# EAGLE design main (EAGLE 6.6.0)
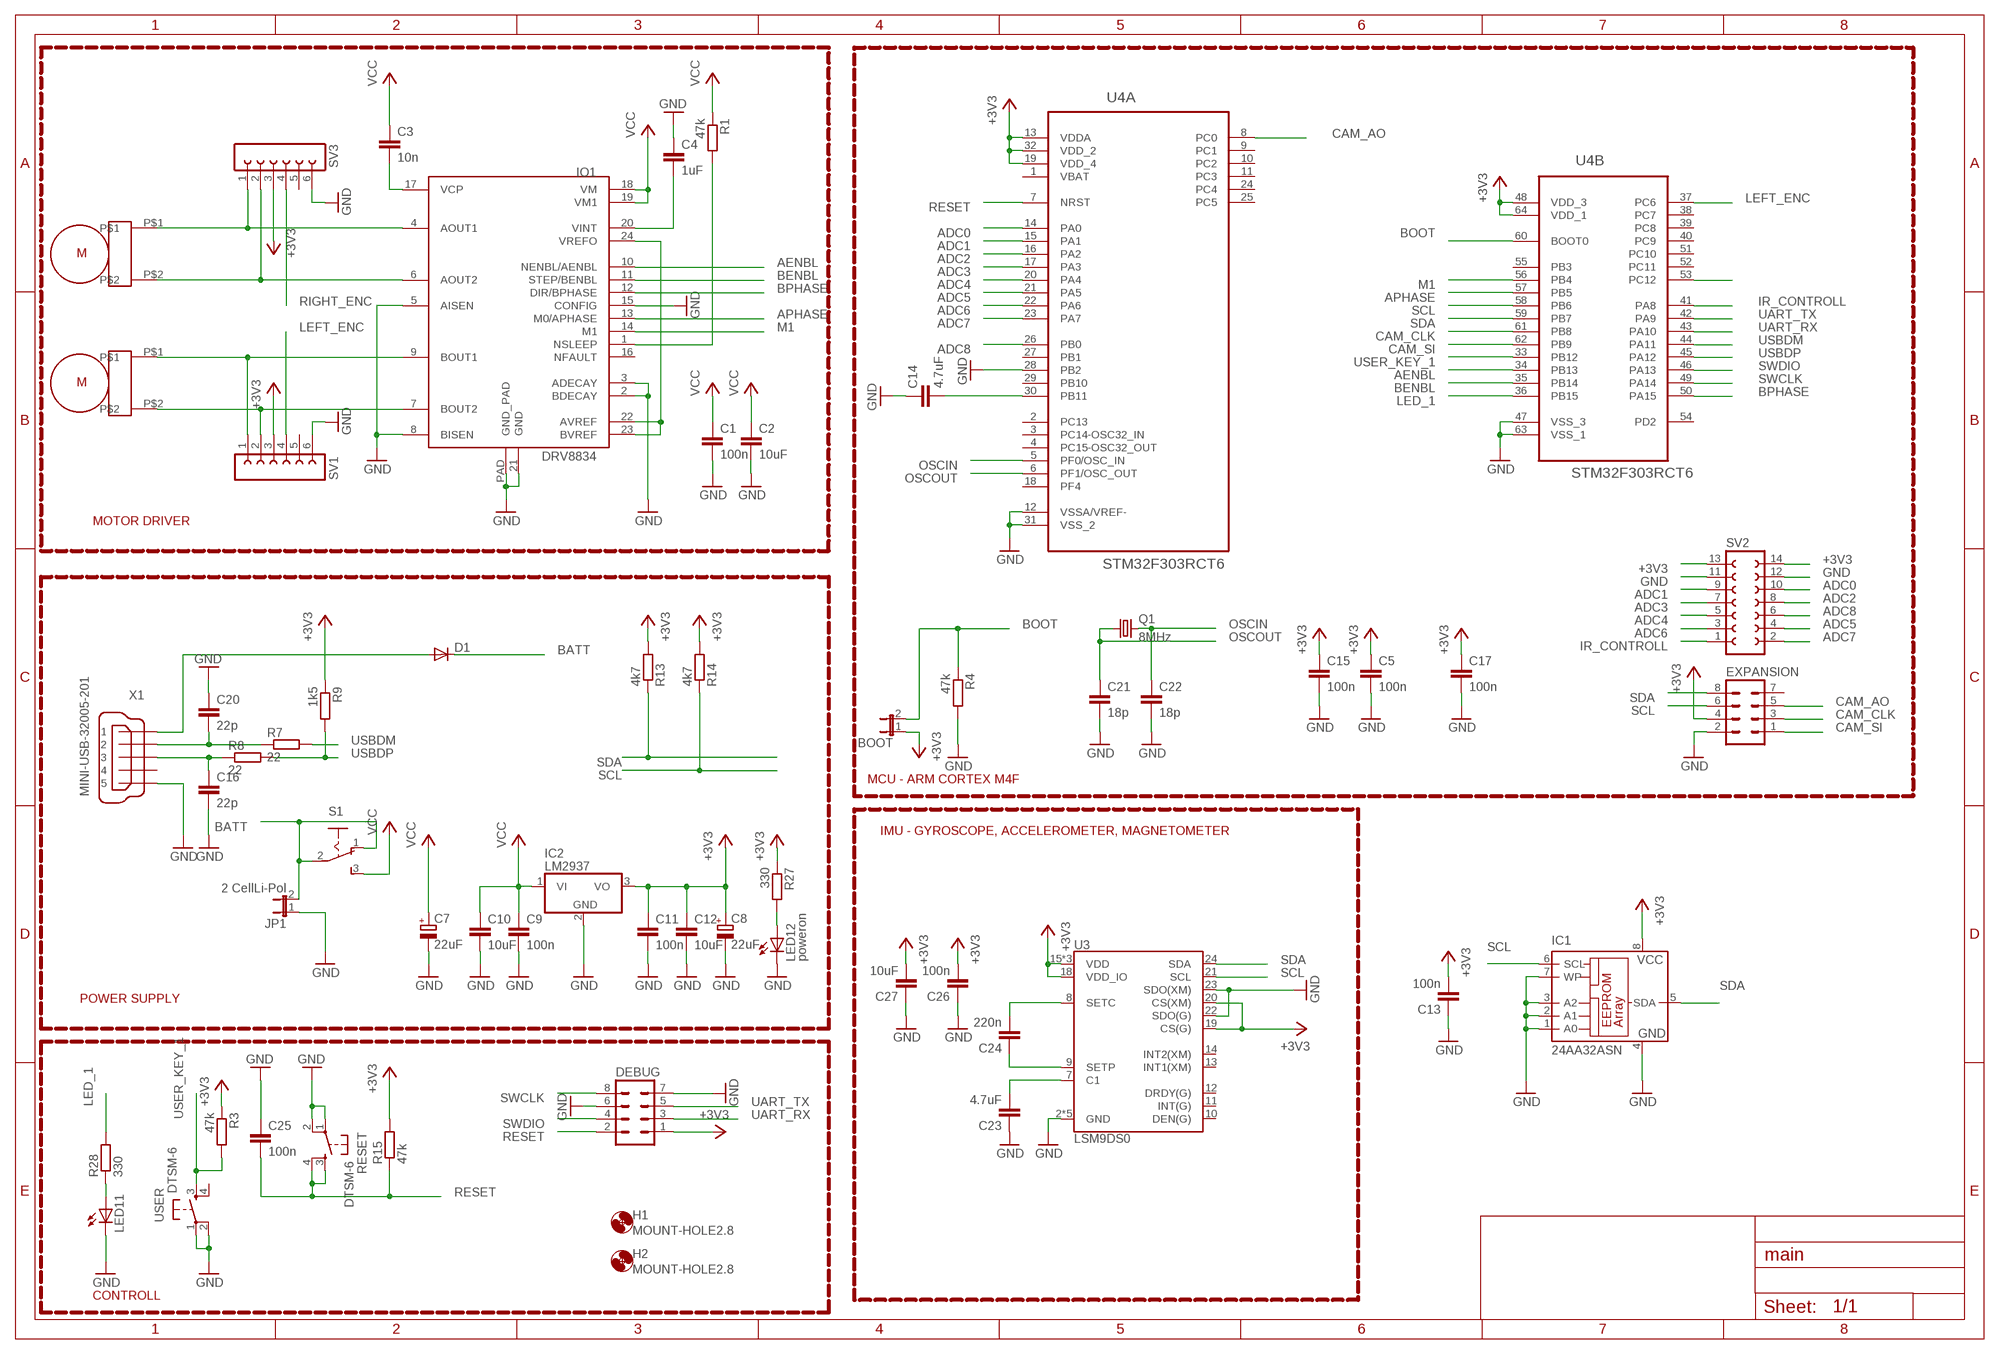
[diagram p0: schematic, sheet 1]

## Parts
BOOT  JP1E  [JP1]
C1  100n  C-EUC1206  [C1206]
C2  10uF  C-EUC1206  [C1206]
C3  10n  C-EUC1206  [C1206]
C4  1uF  C-EUC1206  [C1206]
C5  100n  C-EUC0805  [C0805]
C7  22uF  CPOL-EU153CLV-0505  [153CLV-0505]
C8  22uF  CPOL-EU153CLV-0505  [153CLV-0505]
C9  100n  C-EUC0805  [C0805]
C10  10uF  C-EUC0805  [C0805]
C11  100n  C-EUC0805  [C0805]
C12  10uF  C-EUC0805  [C0805]
C13  100n  C-EUC0805  [C0805]
C14  4.7uF  C-EUC0805  [C0805]
C15  100n  C-EUC0805  [C0805]
C16  22p  C-EUC0805  [C0805]
C17  100n  C-EUC0805  [C0805]
C20  22p  C-EUC0805  [C0805]
C21  18p  C-EUC0805  [C0805]
C22  18p  C-EUC0805  [C0805]
C23  4.7uF  C-EUC0805  [C0805]
C24  220n  C-EUC0805  [C0805]
C25  100n  C-EUC0805  [C0805]
C26  100n  C-EUC0805  [C0805]
C27  10uF  C-EUC0805  [C0805]
D1  DIODE-SMB  [SMB]
DEBUG  MA04-2  [MA04-2]
EXPANSION  MA04-2  [MA04-2]
H1  MOUNT-HOLE2.8  [2,8]
H2  MOUNT-HOLE2.8  [2,8]
IC1  24AA32ASN  [SO-08]
IC2  LM2937  [TO263-3]
IO1  DRV8834  [DRV8834_PCK]
JP1  2 CellLi-Pol  JP1E  [JP1]
LED11  LEDCHIPLED_1206  [CHIPLED_1206]
LED12  poweron  LEDCHIPLED_1206  [CHIPLED_1206]
Q1  8MHz  CRYSTALCTS406  [CTS406]
R1  47k  R-EU_M1206  [M1206]
R3  47k  R-EU_M0805  [M0805]
R4  47k  R-EU_M0805  [M0805]
R7  22  R-EU_M0805  [M0805]
R8  22  R-EU_M0805  [M0805]
R9  1k5  R-EU_M0805  [M0805]
R13  4k7  R-EU_M0805  [M0805]
R14  4k7  R-EU_M0805  [M0805]
R15  47k  R-EU_M0805  [M0805]
R27  330  R-EU_M0805  [M0805]
R28  330  R-EU_M0805  [M0805]
RESET  DTSM-6  [DTSM-6]
S1  255SB  [255SB]
SV1  FE06-1  [FE06]
SV2  FE07-2  [FE07-2]
SV3  FE06-1  [FE06]
U3  LSM9DS0  [LGA-24]
U4  STM32F303RCT6  [QFP50P1200X1200X160-64N]
U$1  MICRO_METAL_GEAR_MOTOR  [MICRO_METAL_GEAR_MOTOR]
U$2  MICRO_METAL_GEAR_MOTOR  [MICRO_METAL_GEAR_MOTOR]
USER  DTSM-6  [DTSM-6]
X1  MINI-USB-32005-201  [32005-201]

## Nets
+3V3: BOOT.1 C5.1 C8.+ C11.1 C12.1 C13.2 C15.1 C17.1 C26.2 C27.2 DEBUG.1 EXPANSION.4 IC1.8(VCC) IC2.3(VO) R3.1 R9.1 R13.2 R14.2 R15.2 R27.1 SV1.3 SV2.13 SV2.14 SV3.3 U3.15(VDD) U3.16(VDD) U3.17(VDD) U3.18(VDD_IO) U3.19(CS(G)) U3.20(CS(XM)) U4.13(A:VDDA) U4.19(A:VDD_4) U4.32(A:VDD_2) U4.48(B:VDD_3) U4.64(B:VDD_1)
ADC0: SV2.10 U4.14(A:PA0)
ADC1: SV2.9 U4.15(A:PA1)
ADC2: SV2.8 U4.16(A:PA2)
ADC3: SV2.7 U4.17(A:PA3)
ADC4: SV2.5 U4.20(A:PA4)
ADC5: SV2.4 U4.21(A:PA5)
ADC6: SV2.3 U4.22(A:PA6)
ADC7: SV2.2 U4.23(A:PA7)
ADC8: SV2.6 U4.26(A:PB0)
AENBL: IO1.10(NENBL/AENBL) U4.34(B:PB13)
APHASE: IO1.13(M0/APHASE) U4.57(B:PB5)
BATT: D1.C JP1.2 S1.1(O) S1.2(P)
BENBL: IO1.11(STEP/BENBL) U4.35(B:PB14)
BOOT: BOOT.2 R4.1 U4.60(B:BOOT0)
BPHASE: IO1.12(DIR/BPHASE) U4.50(B:PA15)
CAM_AO: EXPANSION.5 U4.8(A:PC0)
CAM_CLK: EXPANSION.3 U4.61(B:PB8)
CAM_SI: EXPANSION.1 U4.62(B:PB9)
GND: C1.2 C2.2 C4.1 C5.2 C7.- C8.- C9.2 C10.2 C11.2 C12.2 C13.1 C14.1 C15.2 C16.2 C17.2 C20.1 C21.2 C22.2 C23.1 C25.1 C26.1 C27.1 DEBUG.6 DEBUG.7 EXPANSION.2 IC1.1(A0) IC1.2(A1) IC1.3(A2) IC1.4(GND) IC1.7(WP) IC2.2(GND) IO1.2(BDECAY) IO1.3(ADECAY) IO1.5(AISEN) IO1.8(BISEN) IO1.15(CONFIG) IO1.21(GND) IO1.PAD(GND_PAD) JP1.1 LED11.C LED12.C R4.2 RESET.1 RESET.2 SV1.6 SV2.11 SV2.12 SV3.6 U3.2(GND) U3.3(GND) U3.4(GND) U3.5(GND) U3.6(GND) U3.22(SDO(G)) U3.23(SDO(XM)) U4.12(A:VSSA/VREF-) U4.28(A:PB2) U4.31(A:VSS_2) U4.47(B:VSS_3) U4.63(B:VSS_1) USER.1 USER.2 X1.5
IR_CONTROLL: SV2.1 U4.41(B:PA8)
LED_1: R28.2 U4.36(B:PB15)
LEFT_ENC: SV1.4 U4.37(B:PC6)
M1: IO1.14(M1) U4.56(B:PB4)
N$1: IO1.4(AOUT1) SV3.1 U$1.P$1
N$2: IO1.6(AOUT2) SV3.2 U$1.P$2
N$3: IO1.9(BOUT1) SV1.1 U$2.P$1
N$4: IO1.7(BOUT2) SV1.2 U$2.P$2
N$5: C3.2 IO1.17(VCP)
N$6: C23.2 U3.7(C1)
N$7: C24.2 U3.8(SETC)
N$8: IO1.22(AVREF) IO1.23(BVREF) IO1.24(VREFO)
N$9: IO1.1(NSLEEP) R1.2
N$13: C24.1 U3.9(SETP)
N$15: C14.2 U4.30(A:PB11)
N$22: C4.2 IO1.20(VINT)
N$23: LED12.A R27.2
N$33: LED11.A R28.1
N$55: C20.2 R7.1 X1.2
N$56: C16.1 R8.1 X1.3
N$57: D1.A X1.1
OSCIN: C22.1 Q1.3 U4.5(A:PF0/OSC_IN)
OSCOUT: C21.1 Q1.1 U4.6(A:PF1/OSC_OUT)
RESET: C25.2 DEBUG.2 R15.1 RESET.3 RESET.4 U4.7(A:NRST)
RIGHT_ENC: SV3.4 U4.53(B:PC12)
SCL: EXPANSION.6 IC1.6(SCL) R14.1 U3.21(SCL) U4.58(B:PB6)
SDA: EXPANSION.8 IC1.5(SDA) R13.1 U3.24(SDA) U4.59(B:PB7)
SWCLK: DEBUG.8 U4.49(B:PA14)
SWDIO: DEBUG.4 U4.46(B:PA13)
UART_RX: DEBUG.3 U4.43(B:PA10)
UART_TX: DEBUG.5 U4.42(B:PA9)
USBDM: R7.2 U4.44(B:PA11)
USBDP: R8.2 R9.2 U4.45(B:PA12)
USER_KEY_1: R3.2 U4.33(B:PB12) USER.3
VCC: C1.1 C2.1 C3.1 C7.+ C9.1 C10.1 IC2.1(VI) IO1.18(VM) IO1.19(VM1) R1.1 S1.3(S)
Unconnected: EXPANSION.7 IO1.16(NFAULT) SV1.5 SV3.5 U3.10(DEN(G)) U3.11(INT(G)) U3.12(DRDY(G)) U3.13(INT1(XM)) U3.14(INT2(XM)) U4.2(A:PC13) U4.3(A:PC14-OSC32_IN) U4.4(A:PC15-OSC32_OUT) U4.9(A:PC1) U4.10(A:PC2) U4.11(A:PC3) U4.18(A:PF4) U4.24(A:PC4) U4.25(A:PC5) U4.27(A:PB1) U4.29(A:PB10) U4.38(B:PC7) U4.39(B:PC8) U4.40(B:PC9) U4.51(B:PC10) U4.52(B:PC11) U4.54(B:PD2) U4.55(B:PB3) USER.4 X1.4

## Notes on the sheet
- MOTOR DRIVER
- MCU - ARM CORTEX M4F
- IMU - GYROSCOPE, ACCELEROMETER, MAGNETOMETER
- POWER SUPPLY
- CONTROLL

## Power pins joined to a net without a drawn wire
VBAT: U4.1(A:VBAT)

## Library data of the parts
BOOT JP1 = jumper:JP1E: JUMPER
C1-C5 C9-C17 C20-C27 = resistor:C-EU: CAPACITOR, European symbol
C7 C8 = resistor:CPOL-EU: POLARIZED CAPACITOR, European symbol
D1 = diode:DIODE-: DIODE
DEBUG EXPANSION = con-lstb:MA04-2: PIN HEADER; OC_FARNELL: unknown; OC_NEWARK: unknown
H1 H2 = holes:MOUNT-HOLE: MOUNTING HOLE with drill center marker
IC1 = microchip:24*: Serial EEPROM I2C; MF: MICROCHIP; MPN: 24AA32A-I/SN; OC_FARNELL: 1617659; OC_NEWARK: 83C5815
IC2 = linear:LM2937: LM2937-2.5, LM2937-3.3 400mA and 500mA Voltage Regulators Source: http://cache.national.com/ds/LM/LM2937-2.5.pdf
IO1 = yellow_car:DRV8834
LED11 LED12 = led:LED: LED
Q1 = crystal:CRYSTAL: CRYSTAL; OC_FARNELL: unknown; OC_NEWARK: unknown
R1 R3 R4 R7-R9 R13-R15 R27 R28 = resistor:R-EU_: RESISTOR, European symbol
RESET USER = switch-tact:DTSM-6
S1 = switch:255SB: SLIDING SWITCH Distributor Buerklin, 11G810
SV1 SV3 = con-lsta:FE06-1: FEMALE HEADER; OC_FARNELL: unknown; OC_NEWARK: unknown
SV2 = con-lsta:FE07-2: FEMALE HEADER; OC_FARNELL: unknown; OC_NEWARK: unknown
U3 = SparkFun-DigitalIC:LSM9DS0: LSM9DS0 3D Accelerometer, 3D Gyroscope, 3D Magnetomter Features: 3 acceleration channels, 3 angular rate channels, 3 magnetic field channels ±2/±4/±6/±8/±16 g linear acceleration full scale ±2/±4/±8/±12 gauss magnetic full scale ±245/±500/±2000 dps angular rate full scale 16-bit data output SPI /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
U4 = my_parts:STM32F303RCT6: ARM Cortex-M4 32b MCU+FPU,LQFP-64; MPN: STM32F303RCT6; OC_FARNELL: 2215112; OC_NEWARK: 46W2193; PACKAGE: LQFP-64; SUPPLIER: STMICROELECTRONICS
U$1 U$2 = pololu:MICRO_METAL_GEAR_MOTOR
X1 = con-cypressindustries:MINI-USB-: MINI USB-B Conector Source: www.cypressindustries.com; OC_FARNELL: unknown; OC_NEWARK: unknown

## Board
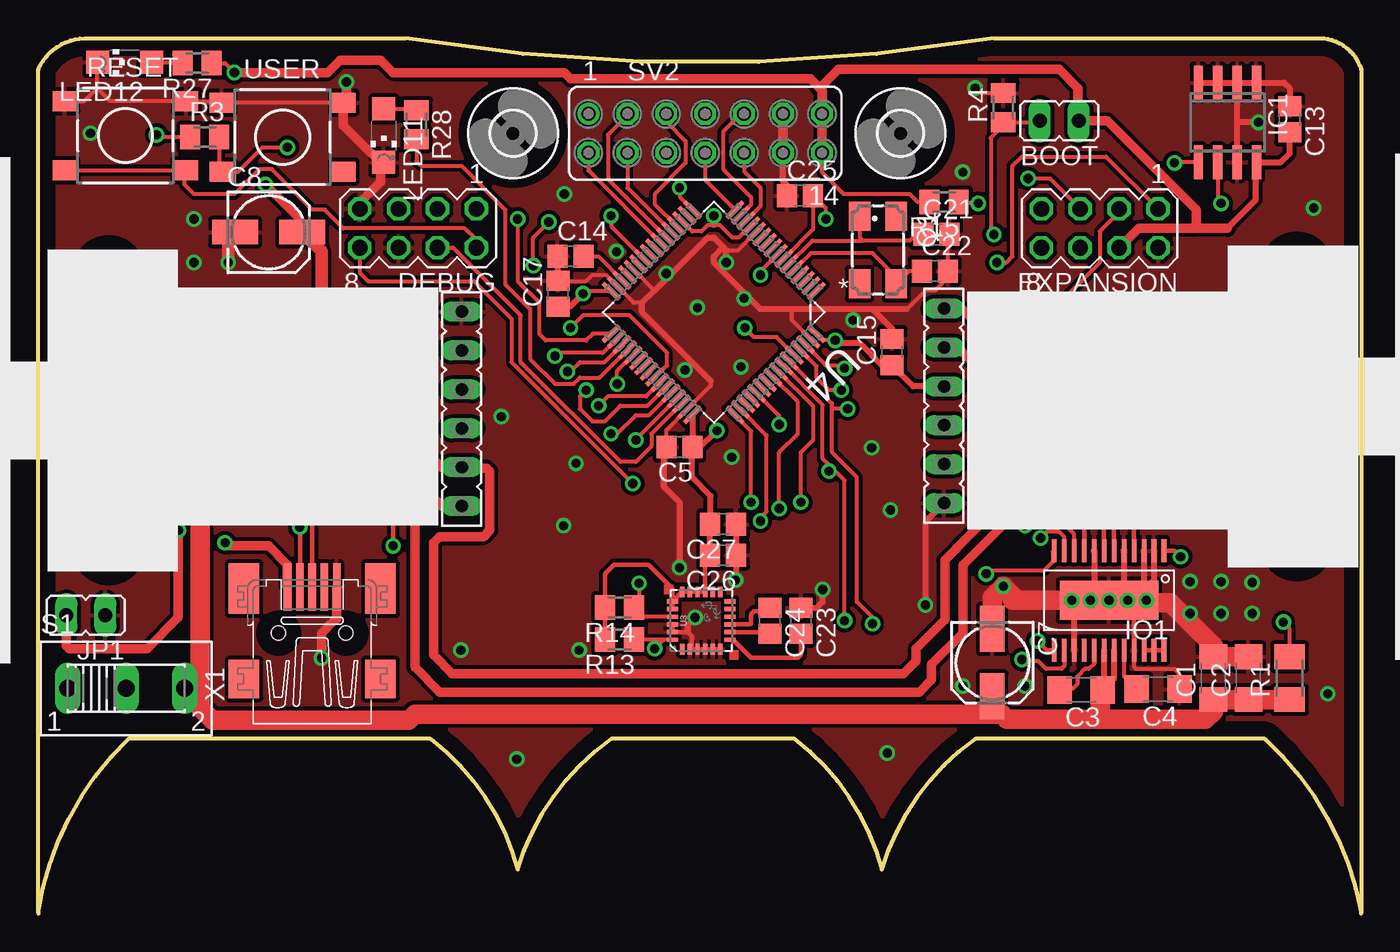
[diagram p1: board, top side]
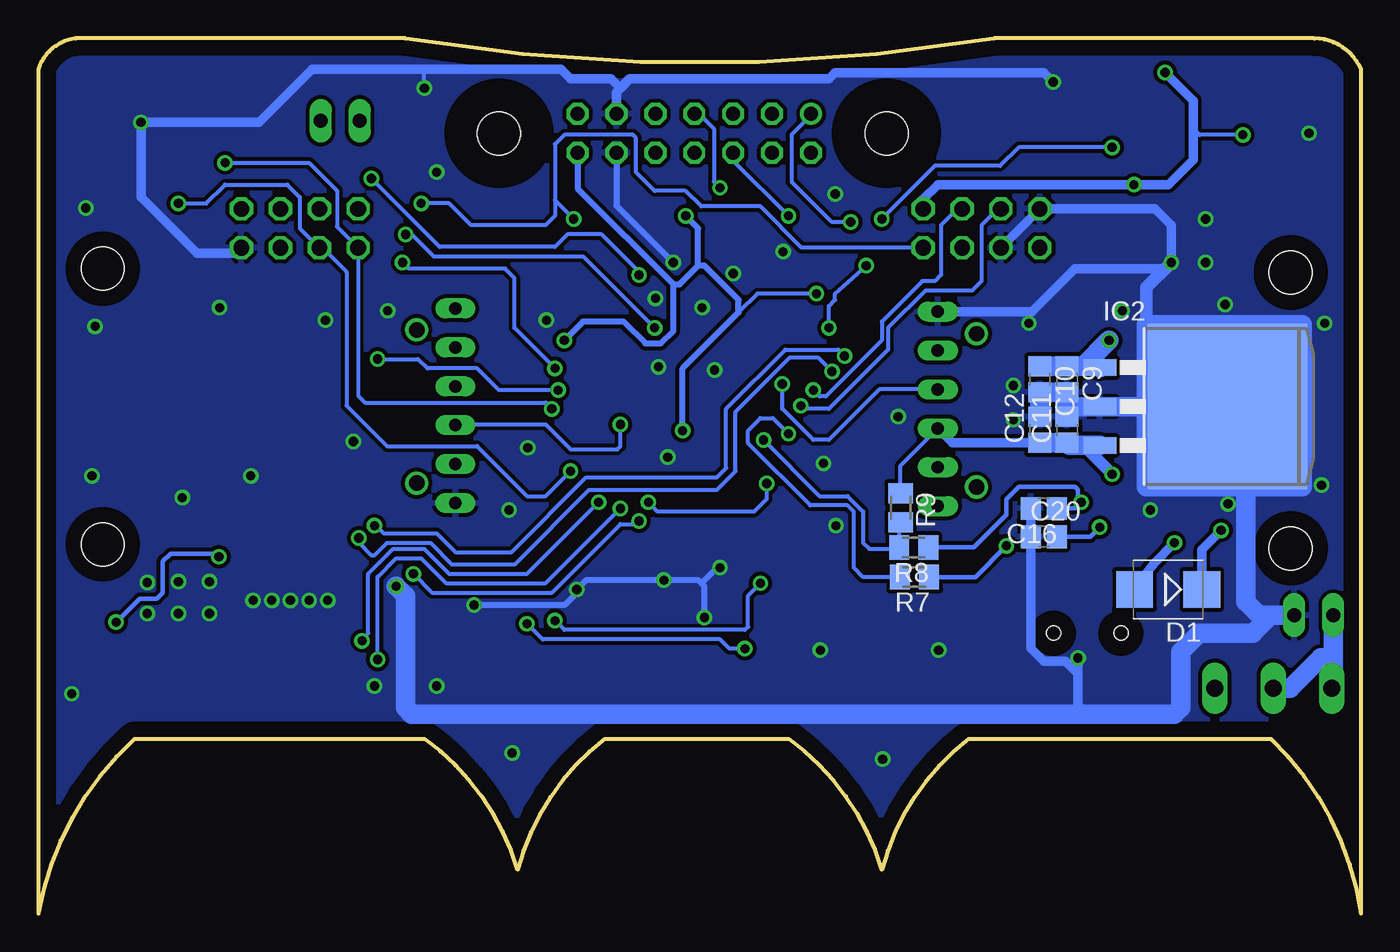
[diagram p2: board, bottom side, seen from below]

Size 86.36 x 57.1 mm. Coordinates in mm from the lower left corner, seen from the top.
Outline: 3.05,57.1 23.98,57.1 arc19 62.38,57.1 83.92,57.1 arc-66 86.36,55.07 86.36,0 arc38 80.06,11.38 61.16,11.38 arc38 55.07,2.85 arc38 49.38,11.38 37.39,11.38 arc38 31.29,2.85 arc38 25.6,11.38 5.89,11.38 arc38 0,0 0,55.07 arc-66 3.05,57.1
Copper layers (1*16): Top 0.035mm / dielectric 1.5mm / Bottom 0.035mm
Design rules "default *": minimum track width 10mil, minimum drill 24mil, track to track 10mil, track to pad 10mil, pad to pad 10mil, via to via 10mil, smd to smd 10mil, copper to edge 40mil, drill to drill 8mil, minimum pad ring 10mil, minimum via ring 8mil, stop-mask expansion 4mil, vias tented up to drill 0mil, thermal gap 10mil

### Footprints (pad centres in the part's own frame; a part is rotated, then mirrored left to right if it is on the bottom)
JP1 = drill 0.914 long: 1 0,-1.27; 2 0,1.27
C1206 = smd 1.6 x 1.8: 1 -1.4,0; 2 1.4,0
C0805 = smd 1.3 x 1.5: 1 -0.85,0; 2 0.85,0
153CLV-0505 = smd 3 x 1.6: + 2.2,0; - -2.2,0
SMB = smd 2.4 x 2.4: A 2.2,0; C -2.2,0
MA04-2 = drill 1.016 octagon: 1 -3.81,-1.27; 2 -3.81,1.27; 3 -1.27,-1.27; 4 -1.27,1.27; 5 1.27,-1.27; 6 1.27,1.27; 7 3.81,-1.27; 8 3.81,1.27
2,8 = hole 2.8: 0,0
SO-08 = smd 0.6 x 2.2: 1 -1.905,-2.6; 2 -0.635,-2.6; 3 0.635,-2.6; 4 1.905,-2.6; 5 1.905,2.6; 6 0.635,2.6; 7 -0.635,2.6; 8 -1.905,2.6
TO263-3 = smd 1.067 x 2.159: 1 -2.54,-5.791; 2 0,-5.791; 3 2.54,-5.791 | smd 10.8 x 10.41: TAB 0,2.54
DRV8834_PCK = smd 0.3 x 1.5: 1 -3.575,-3.25; 2 -2.925,-3.25; 3 -2.275,-3.25; 4 -1.625,-3.25; 5 -0.975,-3.25; 6 -0.325,-3.25; 7 0.325,-3.25; 8 0.975,-3.25; 9 1.625,-3.25; 10 2.275,-3.25; 11 2.925,-3.25; 12 3.575,-3.25; 13 3.575,3.25; 14 2.925,3.25; 15 2.275,3.25; 16 1.625,3.25; 17 0.975,3.25; 18 0.325,3.25; 19 -0.325,3.25; 20 -0.975,3.25; 21 -1.625,3.25; 22 -2.275,3.25; 23 -2.925,3.25; 24 -3.575,3.25 | smd 6.452 x 2.54: PAD 0,0
CHIPLED_1206 = smd 1.5 x 1.5: A 0,-1.75; C 0,1.75
CTS406 = smd 1.9 x 1.4: 1 -2.2,-1.2; 2 2.2,-1.2; 3 2.2,1.2; 4 -2.2,1.2
M1206 = smd 1.6 x 2: 1 -1.4,0; 2 1.4,0
M0805 = smd 1.3 x 1.6: 1 -0.95,0; 2 0.95,0
DTSM-6 = smd 1.55 x 1.3: 1 -3.975,2.25; 2 3.975,2.25; 3 -3.975,-2.25; 4 3.975,-2.25
255SB = drill 1.118 long: 1 -3.81,0; 2 0,0; 3 3.81,0
FE06 = drill 0.813 long: 1 -6.35,0; 2 -3.81,0; 3 -1.27,0; 4 1.27,0; 5 3.81,0; 6 6.35,0
FE07-2 = drill 0.914: 1 -7.62,1.27 | drill 0.914 octagon: 2 -7.62,-1.27; 3 -5.08,1.27; 4 -5.08,-1.27; 5 -2.54,1.27; 6 -2.54,-1.27; 7 0,1.27; 8 0,-1.27; 9 2.54,1.27; 10 2.54,-1.27; 11 5.08,1.27; 12 5.08,-1.27; 13 7.62,1.27; 14 7.62,-1.27
LGA-24 = smd 0.7 x 0.29: 1 -1.875,1.25; 2 -1.875,0.75; 3 -1.875,0.25; 4 -1.875,-0.25; 5 -1.875,-0.75; 6 -1.875,-1.25; 13 1.875,-1.25; 14 1.875,-0.75; 15 1.875,-0.25; 16 1.875,0.25; 17 1.875,0.75; 18 1.875,1.25 | smd 0.29 x 0.7: 7 -1.25,-1.875; 8 -0.75,-1.875; 9 -0.25,-1.875; 10 0.25,-1.875; 11 0.75,-1.875; 12 1.25,-1.875; 19 1.25,1.875; 20 0.75,1.875; 21 0.25,1.875; 22 -0.25,1.875; 23 -0.75,1.875; 24 -1.25,1.875
QFP50P1200X1200X160-64N = smd 1.473 x 0.279: 1 -5.715,3.759; 2 -5.715,3.251; 3 -5.715,2.743; 4 -5.715,2.261; 5 -5.715,1.753; 6 -5.715,1.245; 7 -5.715,0.762; 8 -5.715,0.254; 9 -5.715,-0.254; 10 -5.715,-0.762; 11 -5.715,-1.245; 12 -5.715,-1.753; 13 -5.715,-2.261; 14 -5.715,-2.743; 15 -5.715,-3.251; 16 -5.715,-3.759; 33 5.715,-3.759; 34 5.715,-3.251; 35 5.715,-2.743; 36 5.715,-2.261; 37 5.715,-1.753; 38 5.715,-1.245; 39 5.715,-0.762; 40 5.715,-0.254; 41 5.715,0.254; 42 5.715,0.762; 43 5.715,1.245; 44 5.715,1.753; 45 5.715,2.261; 46 5.715,2.743; 47 5.715,3.251; 48 5.715,3.759 | smd 0.279 x 1.473: 17 -3.759,-5.715; 18 -3.251,-5.715; 19 -2.743,-5.715; 20 -2.261,-5.715; 21 -1.753,-5.715; 22 -1.245,-5.715; 23 -0.762,-5.715; 24 -0.254,-5.715; 25 0.254,-5.715; 26 0.762,-5.715; 27 1.245,-5.715; 28 1.753,-5.715; 29 2.261,-5.715; 30 2.743,-5.715; 31 3.251,-5.715; 32 3.759,-5.715; 49 3.759,5.715; 50 3.251,5.715; 51 2.743,5.715; 52 2.261,5.715; 53 1.753,5.715; 54 1.245,5.715; 55 0.762,5.715; 56 0.254,5.715; 57 -0.254,5.715; 58 -0.762,5.715; 59 -1.245,5.715; 60 -1.753,5.715; 61 -2.261,5.715; 62 -2.743,5.715; 63 -3.251,5.715; 64 -3.759,5.715
MICRO_METAL_GEAR_MOTOR = drill 1: P$1 -5,1; P$2 5,1 | hole 2.8: -9,21.5; 9,21.5
32005-201 = smd 3.1 x 0.5: 1 3,1.6; 2 3,0.8; 3 3,0; 4 3,-0.8; 5 3,-1.6 | smd 2.5 x 2: M1 -3,-4.45; M2 -3,4.45 | smd 3.3 x 2: M3 2.9,4.45; M4 2.9,-4.45 | hole 0.9: 0,2.2; 0,-2.2

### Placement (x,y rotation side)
BOOT  66.65,51.71 90 top
C1  76.71,15.34 90 top
C2  78.99,15.34 90 top
C3  68.07,14.58 180 top
C4  73.1,14.63 180 top
C5  41.86,30.43 180 top
C7  62.28,16.36 270 top
C8  15.04,44.45 0 top
C9  19.2,34.85 270 bottom
C10  20.98,34.85 270 bottom
C11  19.2,31.55 90 bottom
C12  20.98,31.55 90 bottom
C13  81.69,51.82 270 top
C14  34.75,42.88 0 top
C15  55.73,36.63 90 top
C16  20.73,26.42 180 bottom
C17  33.93,40.44 90 top
C20  20.73,24.59 0 bottom
C21  58.62,44.3 0 top
C22  58.52,41.91 0 top
C23  49.78,19.1 270 top
C24  47.75,19.1 270 top
C25  49.73,46.84 0 top
C26  44.7,23.37 180 top
C27  44.7,25.4 180 top
D1  12.6,21.13 180 bottom
DEBUG  24.79,44.7 180 top
EXPANSION  69.29,44.7 180 top
H1  30.99,50.9 0 top
H2  56.29,50.9 0 top
IC1  77.62,51.61 180 top
IC2  11.28,33.07 270 bottom
IO1  69.9,20.42 180 top
JP1  3.1,19.46 90 top
LED11  22.56,50.75 180 top
LED12  5.64,55.52 90 top
Q1  54.81,43.28 270 top
R1  81.69,15.34 90 top
R3  10.87,50.65 0 top
R4  62.99,52.58 90 top
R7  29.16,21.95 180 bottom
R8  29.21,23.88 180 bottom
R9  30.07,26.47 270 bottom
R13  37.95,17.88 180 top
R14  37.95,19.96 180 top
R15  59.13,46.43 180 top
R27  10.36,55.47 180 top
R28  24.69,51.46 270 top
RESET  5.69,50.75 0 top
S1  5.74,14.68 0 top
SV1  27.64,32.92 90 top
SV2  43.54,50.9 0 top
SV3  59.13,33.12 270 top
U3  43.28,19.1 90 top
U4  44.09,39.22 225 top
U$1  60.66,33.07 270 top
U$2  26.11,32.82 90 top
USER  15.95,50.65 0 top
X1  17.88,18.29 90 top

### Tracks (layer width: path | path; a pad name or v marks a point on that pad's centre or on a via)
+3V3  (via drill 0.6)
  Top 0.254: R27.1 12.19,55.47 v12.8,54.86 | R3.1 7.87,50.65 v7.72,50.8 | C5.1 U4.48 | U4.13 46.48,44.86 45.72,44.09 45.31,44.09 44.5,44.91 44.09,44.91 43.69,44.91 43.28,44.5 42.69,44.5 U4.19 | R15.2 57.4,46.43 56.9,46.94 52.58,46.94 51.16,48.36 SV2.14 | U4.32 35.72,40.6 v35.56,40.44 | v52.02,37.39 51.24,37.39 U4.64
  Top 0.305: U3.20 U3.19 | U3.19 U3.18 U3.17 U3.16 U3.15 43.53,23.25 C26.2 | U3.19 41.41,21.18 39.83,22.76 37.59,22.76 36.98,22.15 36.98,19.98 R14.2 R13.2
  Top 0.406: C26.2 C27.2 43.89,25.44 43.89,27.23 42.67,28.45 42.67,30.28 | C13.2 81.69,49.58 81.12,49.01 IC1.8 79.45,48.94 79.45,46.53 77.62,44.7 | 42.67,30.28 42.67,30.39 C5.1 | U4.48 42.71,30.32 42.67,30.28 | 42.67,30.28 43.08,30.28 v44.3,31.5 | v44.09,45.52 44.09,44.91 | C17.1 34.71,39.59 v35.56,40.44 | SV3.3 57.11,34.39 C15.1 55.05,35.78 53.64,37.19 52.22,37.19 v52.02,37.39
  Top 0.61: C8.+ 17.07,44.62 17.07,45.31 v14.83,47.55 | v12.8,54.86 18.9,54.86 19.71,55.68 22.35,55.68 23.16,54.86 34.34,54.86 34.75,54.46 50.39,54.46 51.21,53.65 51.21,52.22 SV2.13 SV2.14 51.16,54 52.22,55.07 66.65,55.07 67.87,53.85 67.87,51.77 BOOT.1 69.8,51.71 75.59,45.92 75.59,44.91 75.39,44.7 | 75.39,44.7 71.83,44.7 EXPANSION.4 | 77.62,44.7 75.39,44.7
  Top 0.813: v16.26,28.65 16.26,34.54 18.49,36.78 18.49,43.2 C8.+
  Bottom 0.254: v7.72,50.8 10.57,50.8 10.97,51.21 | v35.56,40.44 39.42,40.44 40.64,39.22 | R9.1 30.07,29.21 SV1.3
  Bottom 0.406: SV2.14 51.16,47.3 44.91,41.05 | 44.91,41.05 44.5,41.05 43.28,42.27 | v44.3,31.5 44.3,35.56 40.64,39.22 40.64,40.03 42.88,42.27 43.28,42.27 | 43.28,42.27 43.28,44.7 v44.09,45.52 | 44.91,41.05 44.91,38 45.72,37.19 46.74,37.19 48.16,38.61 50.8,38.61 v52.02,37.39
  Bottom 0.61: DEBUG.1 28.6,46.58 27.63,47.55 v14.83,47.55 12.6,47.55 10.97,49.17 10.97,51.21 10.97,53.04 v12.8,54.86 | C12.1 26.68,30.7 SV1.3
  Bottom 0.813: C12.1 18.3,30.7 v16.26,28.65
  Bottom 1.27: IC2.3 19.04,30.53 C11.1 C12.1
ADC0
  Top 0.254: SV2.10 46.08,48.41 47.14,47.35 47.14,46.15 U4.14
ADC1
  Top 0.254: SV2.9 45.87,52.17 44.7,51 44.7,48.57 46.53,46.74 46.53,46.25 U4.15
ADC2
  Top 0.254: SV2.8 43.54,47.86 U4.16
ADC3  (via drill 0.6)
  Top 0.254: v41.86,47.35 41.86,46.77 U4.17
  Bottom 0.254: SV2.7 43.23,52.17 42.27,51.21 42.27,47.75 v41.86,47.35
ADC4
  Top 0.254: SV2.5 41,51.66 42.27,50.39 42.27,48.97 40.23,46.94 40.23,46.28 U4.20
ADC5
  Top 0.254: SV2.4 38.46,47.34 U4.21
ADC6
  Top 0.254: SV2.3 38.46,52.07 37.19,50.8 37.19,47.89 U4.22
ADC7
  Top 0.254: SV2.2 35.92,48.47 U4.23
ADC8  (via drill 0.6)
  Top 0.254: v37.39,45.52 37.39,44.85 U4.26
  Bottom 0.254: SV2.6 41,49.12 v37.39,45.52
AENBL  (via drill 0.6)
  Top 0.254: IO1.10 67.63,24.73 66.85,25.5 64.62,25.5 v64.41,25.3 | U4.34 36.85,36.58 33.93,36.58 v33.73,36.37
  Bottom 0.254: v64.41,25.3 64.31,25.3 63.8,24.79 60.35,24.79 59.13,23.57 55.47,23.57 50.6,28.45 42.06,28.45 41.45,29.06 41.45,32.92 37.59,36.78 34.14,36.78 v33.73,36.37
APHASE  (via drill 0.6)
  Top 0.254: IO1.13 65.84,17.17 v65.23,17.78 | v49.78,26.82 49.78,30.07 50.6,30.89 50.6,33.07 U4.57
  Bottom 0.254: v65.23,17.78 65.23,17.88 64.82,18.29 64.82,22.15 63.2,23.77 61.16,23.77 59.54,22.15 54.46,22.15 v49.78,26.82
BATT  (via drill 0.6)
  Top 0.61: v9.14,24.99 9.14,19.3 7.11,17.27 2.03,17.27 1.83,17.48 JP1.2
  Bottom 0.61: D1.C 10.4,23.74 v9.14,24.99
  Bottom 1.27: JP1.2 1.83,16.66 | 1.83,16.66 1.83,14.78 S1.1 | S1.2 4.62,14.68 2.64,16.66 1.83,16.66
BENBL  (via drill 0.6)
  Top 0.254: IO1.11 66.98,24.57 66.65,24.89 65.84,24.89 v65.43,24.49 | v34.54,35.36 34.75,35.36 35.36,35.97 36.96,35.97 U4.35
  Bottom 0.254: v65.43,24.49 65.43,24.18 64.62,23.37 64.41,23.37 63.6,24.18 60.76,24.18 59.33,22.76 55.27,22.76 50.39,27.64 42.06,27.64 40.84,28.85 40.84,32.72 37.28,36.28 35.47,36.28 v34.54,35.36 34.75,35.56
BOOT  (via drill 0.6)
  Top 0.254: BOOT.2 65.29,51.63 R4.1 62.99,51.41 62.18,50.6 62.18,44.5 v62.38,44.3 | U4.60 48.2,37.59 46.74,37.59 v46.13,38.2
  Bottom 0.254: v46.13,38.2 50.8,42.88 60.55,42.88 61.98,44.3 v62.38,44.3
BPHASE  (via drill 0.6)
  Top 0.254: 66.33,23.55 IO1.12 66.23,23.57 66.23,22.94 65.63,22.35 62.08,22.35 v61.87,22.15 | v47.14,25.6 47.14,25.81 47.55,26.21 47.55,31.17 U4.50
  Bottom 0.254: v61.87,22.15 60.65,20.93 52.83,20.93 48.36,25.4 47.35,25.4 v47.14,25.6
CAM_AO  (via drill 0.6)
  Top 0.254: v64.62,47.96 66.04,47.96 EXPANSION.5 | v47.14,41.66 47.14,41.91 U4.8
  Bottom 0.254: v47.14,41.66 47.14,41.86 49.58,44.3 51.82,44.3 52.63,43.49 60.15,43.49 v64.62,47.96
CAM_CLK  (via drill 0.6)
  Top 0.254: EXPANSION.3 70.56,45.77 69.29,44.5 69.29,42.47 64.21,37.39 v64.21,36.17 | v52.43,34.14 51.61,34.14 50.8,34.95 50.8,35.71 U4.61
  Bottom 0.254: v64.21,36.17 61.57,36.17 60.96,35.56 57.71,35.56 56.29,34.14 v52.43,34.14
CAM_SI  (via drill 0.6)
  Top 0.254: U4.62 50.07,37.1 51.41,35.76 52.43,35.76 v52.63,35.56 | v62.59,42.47 63.2,42.47 63.6,42.88 63.6,48.77 64.21,49.38 69.7,49.38 EXPANSION.1
  Bottom 0.254: v52.63,35.56 55.27,38.2 55.27,41.45 55.88,42.06 62.18,42.06 v62.59,42.47
GND  (via drill 0.6)
  Top 0.254: 72.18,20.46 72.3,20.46 v72.34,20.42 | v67.46,20.42 v68.68,20.42 IO1.PAD 70.31,20.02 | IO1.21 71.53,16.05 71.63,15.95 74.17,15.95 74.42,15.7 74.42,14.71 C4.1 | RESET.1 3.01,53 3.86,53.85 | 3.86,53.85 3.86,55.5 LED12.C | 3.86,53.85 4.71,53 RESET.2 11.87,53 USER.1 USER.2 | C5.2 41.01,31.53 U4.47 43.89,34.42 43.89,34.75 | C14.1 33.9,41.9 34.54,41.25 35.76,41.25 36.17,41.66 37.06,41.66 U4.31 38.89,39.83 39.42,39.83 | C21.2 59.37,44.2 C22.2 59.37,41.49 58.52,40.64 57.91,40.64 56.69,39.42 | R4.2 61.48,53.53 v61.16,53.85 | 44.91,43.28 45.68,43.28 U4.12 | 49.17,39.42 49.17,38.74 U4.63 | U4.28 38.85,42.02 40.23,40.64
  Top 0.305: 70.51,20.22 70.31,20.02 | 71.53,20.42 71.73,20.42 72.83,21.52 | 71.53,20.42 v71.12,20.42 71.04,20.42 70.88,20.58 | 67.97,20.32 68.07,20.42 v68.68,20.42 | 71.53,20.42 | 71.53,19.81 IO1.21 | U3.6 U3.5 U3.4 U3.3 U3.2 42.67,17.37 42.67,18.09 42.41,18.35 U3.23 U3.22
  Top 0.406: 71.73,20.42 71.53,20.22 71.53,19.81 72.18,20.46 IO1.3 | IO1.2 72.83,21.72 71.53,20.42 | IO1.5 70.88,20.58 70.51,20.22 | IO1.15 67.63,19.98 67.97,20.32 | IO1.8 68.93,20.58 69.09,20.42 | C27.1 C26.1 45.55,21.78 v45.52,21.74 | v51.21,21.13 51.21,20.32 50.8,19.91 49.82,19.91 C23.1 | 42.41,18.35 42.41,18.84 v42.88,19.3 | v41.86,22.56 41.86,26.82 40.84,27.84 40.84,30.26 C5.2 | IC1.4 IC1.3 IC1.2 | IC1.2 IC1.1 81.32,54.21 81.69,53.85 C13.1 | IC1.7 78.26,51.61 | 78.26,51.61 IC1.2 | v79.65,51.61 78.26,51.61 | 56.69,39.42 54.46,39.42 | 54.46,39.42 49.17,39.42 47.14,39.42 44.09,42.47 44.09,42.88 44.7,43.49 | 43.89,34.75 39.42,39.22 39.42,39.83 40.23,40.64 43.69,44.09 44.09,44.09 44.7,43.49 | 44.7,43.49 44.91,43.28 v44.91,42.47 | C25.1 48.88,47.48 48.62,47.75 SV2.12 | C17.2 33.93,42.84 C14.1 | C15.2 55.73,38.15 54.46,39.42 | SV3.6 57.91,25.55 v57.91,20.12
  Top 0.61: X1.5 19.48,19.18 19.38,19.18 18.49,18.29 v18.49,16.66 | DEBUG.7 20.98,46.38 22.35,47.75 22.35,48.8 LED11.C 22.32,49 19.91,51.41 19.91,52.89 USER.2 20.12,53.09 v20.12,54.25 | SV2.12 SV2.11
  Top 0.813: v12.4,42.47 12.4,44.01 C8.-
  Top 1.27: 63.6,20.42 v67.46,20.42 | 69.09,20.42 v68.68,20.42 63.91,20.42 v62.99,21.34 62.28,20.63 C7.- | v72.34,20.42 72.49,20.27 73.91,20.27 76.71,17.48 C1.2 C2.2
  Bottom 0.254: v61.16,53.85 61.16,55.07
  Bottom 0.406: v42.88,19.3 42.88,21.34 43.08,21.54 | 43.08,21.54 43.28,21.74 v45.52,21.74 50.6,21.74 v51.21,21.13 51.21,20.93 52.02,20.12 v57.91,20.12 | v41.86,22.56 42.06,22.56 43.08,21.54 | SV2.12 48.62,46.18 v44.91,42.47
  Bottom 0.61: v18.49,16.66 18.49,15.65 | 18.49,15.65 18.49,13.61 17.88,13.01 | C16.2 C20.1 21.58,17.31 20.73,16.46 19.3,16.46 18.49,15.65 | 48.36,53.85 48.62,53.59 SV2.11 | 48.36,53.85 47.75,54.46 34.75,54.46 34.34,54.86 20.73,54.86 v20.12,54.25 | 23.52,43.38 DEBUG.6 DEBUG.7 13.46,45.97 12.4,44.91 v12.4,42.47 12.8,42.06 18.69,42.06 21.49,39.27 SV1.6 | 48.36,53.85 48.97,54.46 51.61,54.46 52.22,55.07 61.16,55.07 68.48,55.07 71.93,51.61 v79.65,51.61 79.65,46.74 76,43.08 73.46,43.08 EXPANSION.2
  Bottom 0.813: 14.02,38.41 14.02,40.84 v12.4,42.47
  Bottom 1.27: v62.99,21.34 62.38,20.73 62.38,13.41 61.98,13.01 17.88,13.01 12.19,13.01 11.79,13.41 11.79,17.07 10.57,18.29 7.06,18.29 5.89,19.46 | JP1.1 5.89,19.46 | 5.89,19.46 6.65,19.46 7.52,20.32 7.52,27.64 7.31,27.84 | 14.02,33.07 IC2.2 19.25,33.07 19.3,33.12 19.3,32.5 C11.2 C9.2 C10.2 C12.2 | 14.02,33.07 14.02,38.41 3.86,38.41 3.86,27.84 7.31,27.84 | 7.31,27.84 14.02,27.84 14.02,33.07
  other vias: 77.22,19.56 75.18,19.56 75.18,21.64 77.22,21.64 69.9,20.42 79.25,19.56 79.25,21.59 72.49,28.55 84.18,14.33 60.35,14.83 10.16,42.47 64.41,14.83 13.77,26.31 2.59,27.94 2.39,38.51 15.6,39.32 22.71,34.44 22.71,32.21 8.89,39.73 8.69,26.72 10.16,45.31 65.79,30.78 54.41,30.38 55.63,26.31 67.61,38.71 63.55,39.32 34.29,25.3 27.58,17.17 3.4,50.9 43.03,39.52 35.1,29.36 30.23,32.41 35.31,17.17 31.24,10.06 55.42,10.46 82.65,38.3 82.85,28.55 74.52,39.52 76.96,27.13 83.26,46.02 53.19,38.71 45.26,29.77 42.21,35.46 46.08,40.13 60.35,48.36 34.34,46.94 21.69,38.51 45.87,35.66 41,41.76 37.74,43.18
  pour Bottom: -4.67,61.57 94.08,61.57 94.08,-3.86 -4.67,-3.86
  pour Top: -3.86,72.54 89.2,72.54 89.2,-5.49 -3.86,-5.49
IR_CONTROLL  (via drill 0.6)
  Top 0.254: U4.41 40.28,35 41.05,35.76 41.05,36.58 38.61,39.01 35.56,39.01 v34.75,38.2 | v32.31,42.27 32.31,44.09 v33.32,45.11
  Bottom 0.254: SV2.1 35.92,52.07 37.19,50.8 37.19,47.75 34.54,45.11 v33.32,45.11 | v34.75,38.2 34.75,39.62 34.34,40.03 34.34,40.44 v32.31,42.27
LED_1
  Top 0.254: R28.2 24.69,49.07 24.99,48.77 27.63,48.77 30.48,45.92 30.48,41.05 32.11,39.42 32.11,36.17 33.73,34.54 34.95,34.54 35.36,34.95 36.63,34.95 U4.36
LEFT_ENC  (via drill 0.6)
  Top 0.254: v37.79,34.54 37.79,35.4 U4.37
  Bottom 0.254: SV1.4 31.45,34.19 34.75,30.89 35.76,30.89 37.79,32.92 v37.79,34.54
M1  (via drill 0.6)
  Top 0.254: IO1.14 66.98,16.13 66.8,15.95 65.79,15.95 65.28,16.46 64.31,16.46 v64.21,16.56 | v48.36,26.42 48.36,30.07 49.58,31.29 49.58,33.37 U4.56
  Bottom 0.254: v64.21,16.56 64.21,21.95 62.99,23.17 61.37,23.17 59.74,21.54 53.24,21.54 v48.36,26.42 48.56,26.21
N$1
  Top 0.305: IO1.4 71.53,25.7
  Top 0.406: 71.53,25.7 71.53,25.71
  Top 0.61: 71.53,25.71 71.53,27.23 69.29,29.46 63.4,29.46 62.99,29.87 62.99,36.73 U$1.P$1 60.25,39.47 SV3.1
N$2
  Top 0.305: IO1.6 70.23,26.4
  Top 0.406: 70.23,26.4 69.09,27.53
  Top 0.61: 69.09,27.53 68.28,28.35 68.25,28.33 61.91,28.33 | 61.91,28.33 U$1.P$2 | 61.91,28.33 61.91,35.02 60.15,36.78 59.28,36.78 SV3.2
N$3
  Top 0.305: IO1.9 68.28,25.5
  Top 0.406: 68.28,25.5 67.56,26.21 67.46,26.31
  Top 0.61: 67.56,26.21 67.16,26.62 64.26,26.62 60.35,22.71 60.35,18.29 58.32,16.26 58.32,15.24 57.51,14.43 26.21,14.43 24.59,16.05 24.59,27.29 U$2.P$1 26.36,26.57 SV1.1
N$4
  Top 0.254: 27.69,29.06 SV1.2
  Top 0.305: IO1.7 69.58,25.42
  Top 0.406: 69.58,25.42 67.67,27.33
  Top 0.61: 67.87,27.13 67.67,27.33 67.46,27.53 63.65,27.53 59.94,23.83 59.94,23.8 59.18,23.04 59.18,19.15 57.3,17.27 57.3,16.46 56.49,15.65 27.03,15.65 25.81,16.87 25.81,24.18 26.21,24.59 29.06,24.59 29.46,24.99 29.46,28.85 29.26,29.06 27.69,29.06 | U$2.P$2 25.15,37.78 25.15,30.28 26.31,29.11 SV1.2
N$5
  Top 0.254: IO1.17 68.93,16.3 68.58,15.95 68.33,15.95 67.82,15.44 67.82,14.94 67.56,14.68 66.77,14.68 C3.2
N$6
  Top 0.305: U3.7 45.34,17.85 46.53,16.66 49.58,16.66 49.78,16.87 C23.2
N$7
  Top 0.305: U3.8 47.65,18.35 C24.2
N$8
  Top 0.305: IO1.24 IO1.23 IO1.22
N$9  (via drill 0.6)
  Top 0.254: R1.2 81.69,18.59 v81.28,19
  Top 0.305: IO1.1 74.17,23.67 v74.57,23.27
  Bottom 0.305: v74.57,23.27 74.78,23.47 77.72,23.47 78.23,22.96 78.23,20.93 78.64,20.52 79.76,20.52 v81.28,19
N$13
  Top 0.305: U3.9 46.49,18.85 46.53,18.9 46.53,19.51 46.74,19.71 47.51,19.71 C24.1
N$15
  Top 0.254: C14.2 36.56,42.88 U4.30
N$22
  Top 0.254: IO1.20 70.88,15.46 C4.2
N$23
  Top 0.254: LED12.A 9.36,55.52 R27.2
N$33
  Top 0.254: LED11.A 24.6,52.5 R28.1
N$55  (via drill 0.6)
  Top 0.305: X1.2 17.08,25.18 v17.07,25.2 17.07,27.64 17.88,28.45 21.74,28.45 23.16,27.03 v23.16,23.98
  Bottom 0.305: C20.2 17.68,24.59 v17.07,25.2 | R7.1 25.2,21.95 v23.16,23.98
N$56  (via drill 0.6)
  Top 0.305: X1.3 17.88,26.42 v18.29,26.82
  Bottom 0.305: C16.1 18.69,26.42 v18.29,26.82 18.49,27.03 18.49,27.64 18.69,27.84 22.35,27.84 23.16,27.03 23.16,26.01 25.3,23.88 R8.1
N$57  (via drill 0.6)
  Top 0.406: 16.26,21.31 X1.1
  Top 0.61: 16.26,21.31 16.26,22.76 15.04,23.98 12.4,23.98 v12.19,24.18
  Bottom 0.61: D1.A 13.58,22.79 v12.19,24.18
OSCIN
  Top 0.254: U4.5 50.43,43.08 54.46,43.08 56.01,41.52 Q1.3 56.84,41.91 C22.1
OSCOUT
  Top 0.254: 53.41,45.48 Q1.1 53.64,45.45 53.64,44.09 53.85,43.89 | U4.6 50.53,43.89 53.85,43.89 | C21.1 57.3,44.3 56.9,43.89 54.86,43.89 53.85,43.89
RESET  (via drill 0.6)
  Top 0.254: RESET.3 RESET.4 9.55,48.39 9.55,47.55 10.16,46.94 12.8,46.94 14.43,48.57 15.24,48.57 17.88,45.92 18.69,45.92 19.91,44.7 27.84,44.7 28.6,43.94 DEBUG.2 | U4.7 50.58,44.63 C25.2 51.41,46.01 v51.41,45.31 | v61.37,46.33 60.18,46.33 R15.1
  Bottom 0.254: DEBUG.2 36.52,43.43 39.22,46.13 43.08,46.13 44.09,47.14 46.13,47.14 47.35,48.36 47.35,50.6 47.55,50.8 52.02,50.8 52.63,50.19 52.63,46.53 | 52.63,46.53 v51.41,45.31 | 52.63,46.53 52.63,45.52 53.24,44.91 58.12,44.91 59.54,46.33 v61.37,46.33
RIGHT_ENC  (via drill 0.6)
  Top 0.254: v48.36,31.9 48.36,32.47 U4.53
  Bottom 0.254: SV3.4 59.08,31.9 53.24,31.9 51.61,30.28 48.56,30.28 48.36,30.48 v48.36,31.9
SCL  (via drill 0.6)
  Top 0.254: IC1.6 76.99,46.56 v77.22,46.33 | v52.63,19.1 52.63,28.25 51.61,29.26 | U4.58 51.21,33.18 51.21,29.67 51.61,29.26 | v39.22,21.54 39.22,20.28 R14.1 39.51,19.35 U3.21 | v51.61,28.85 51.61,29.26
  Bottom 0.254: v77.22,46.33 75.39,46.33 74.17,47.55 70.1,47.55 69.29,46.74 69.29,44.7 EXPANSION.6 68.02,43.23 67.62,43.23 66.24,41.86 66.24,33.12 63.6,30.48 57.71,30.48 54.46,27.23 53.24,27.23 v51.61,28.85 | v52.63,19.1 52.02,18.49 40.23,18.49 40.03,18.69 40.03,20.73 v39.22,21.54
SDA  (via drill 0.6)
  Top 0.254: IC1.5 74.21,49.01 v74.17,48.97 | R13.1 38.93,17.85 U3.24 40.81,17.85 v40.23,17.27 | v54.46,18.9 54.46,19.3 53.44,20.32 53.44,28.45 51.82,30.07 51.82,32.92 | 51.82,32.92 51.82,33.26 U4.59 | v52.83,32.92 51.82,32.92
  Bottom 0.254: v74.17,48.97 68.68,48.97 66.85,47.14 66.85,44.81 EXPANSION.8 65.48,33.78 65.02,33.33 53.24,33.33 v52.83,32.92 | v40.23,17.27 41.25,17.27 41.86,17.88 53.44,17.88 v54.46,18.9
SWCLK  (via drill 0.6)
  Top 0.254: DEBUG.8 20.98,41.81 21.54,41.25 28.45,41.25 30.89,38.81 30.89,35.97 v38.81,28.04 | U4.49 46.53,31.46 v46.53,26.82
  Bottom 0.254: v38.81,28.04 38.81,27.03 39.62,26.21 45.92,26.21 v46.53,26.82
SWDIO
  Top 0.254: DEBUG.4 27.08,43.43 30.48,40.03 30.89,39.62 31.5,39.01 31.5,35.97 38,29.46 39.01,29.46 40.03,30.48 40.03,31.29 41.97,33.24 U4.46
UART_RX  (via drill 0.6)
  Top 0.254: v35.76,34.14 35.36,33.73 35.36,32.92 36.17,32.11 36.98,32.11 38,33.12 39.76,33.12 U4.43
  Bottom 0.254: DEBUG.3 26.36,45.97 27.43,44.91 27.43,41.66 27.84,41.25 28.65,41.25 31.29,38.61 31.29,37.39 34.95,33.73 35.36,33.73 v35.76,34.14
UART_TX  (via drill 0.6)
  Top 0.254: U4.42 39.69,33.73 37.19,33.73 v36.58,33.12
  Bottom 0.254: DEBUG.5 23.72,45.97 24.79,44.91 24.79,41.25 25.4,40.64 28.45,40.64 30.89,38.2 30.89,36.78 34.75,32.92 36.37,32.92 v36.58,33.12
USBDM  (via drill 0.6)
  Top 0.254: v37.39,31.29 37.79,31.29 39.01,32.51 39.87,32.51 U4.44
  Bottom 0.254: R7.2 32.51,21.95 33.12,22.56 33.12,26.21 33.53,26.62 35.97,26.62 40.03,30.68 40.03,31.5 39.22,32.31 38.41,32.31 v37.39,31.29
USBDP  (via drill 0.6)
  Top 0.254: v39.01,30.89 39.01,30.94 U4.45
  Bottom 0.254: v39.01,30.89 35.36,27.23 33.53,27.23 32.51,26.21 32.51,24.18 32.11,23.77 30.26,23.77 R8.2 30.16,25.43 R9.2
  Bottom 0.305: 30.16,25.78 R9.2
USER_KEY_1  (via drill 0.6)
  Top 0.254: R3.2 11.82,48.55 USER.3 13.04,48.4 14.63,49.99 v16.26,49.99 | v31.29,45.31 31.29,41.25 32.71,39.83 32.71,37.8 33.12,37.39 35.76,37.39 36.21,37.83 U4.33
  Bottom 0.254: v16.26,49.99 22.35,49.99 23.57,48.77 27.84,48.77 v31.29,45.31
VCC  (via drill 0.6)
  Top 0.254: C7.+ 62.28,13.11 62.38,13.01
  Top 0.305: 69.58,14.43 C3.1
  Top 0.406: 10.97,20.02 10.67,20.02 10.57,20.12 | IO1.18 69.58,14.68 C3.1 70.23,15.33 IO1.19
  Top 1.27: 69.49,14.3 C3.1 69.34,14.2 69.34,12.9 69.09,12.65 | 69.09,12.65 63.25,12.65 62.89,13.01 62.38,13.01 24.59,13.01 24.18,12.6 11.38,12.6 10.57,13.41 10.57,15.04 | 69.09,12.65 76.2,12.65 76.71,13.16 C1.1 C2.1 R1.1 | S1.3 10.21,14.68 10.57,15.04 | 10.57,15.04 10.57,20.12 10.57,36.17 11.79,37.39 v16.46,37.39
  Bottom 1.27: IC2.1 17.16,35.7 C9.1 C10.1 18.15,35.7 v16.46,37.39
(copper drawn outside any net)
  shapes: Top area x2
